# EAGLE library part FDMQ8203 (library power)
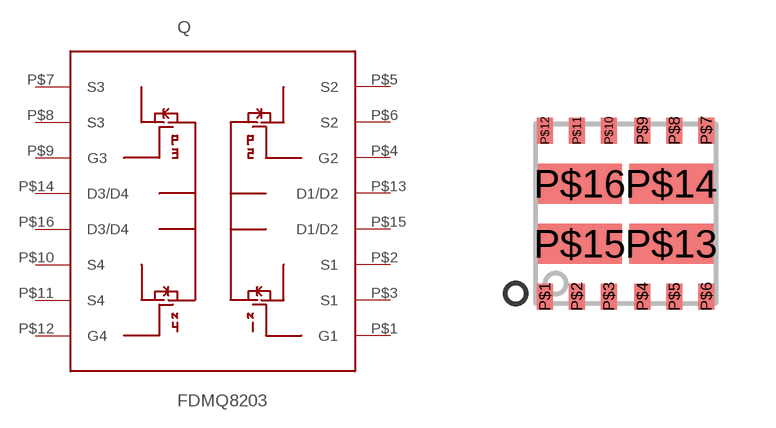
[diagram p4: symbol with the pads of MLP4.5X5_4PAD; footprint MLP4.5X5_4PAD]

Designator prefix Q

## FDMQ8203  [MLP4.5X5_4PAD]
P$1  G1
P$2  S1
P$3  S1
P$4  G2
P$5  S2
P$6  S2
P$7  S3
P$8  S3
P$9  G3
P$10  S4
P$11  S4
P$12  G4
P$13  D1/D2
P$14  D3/D4
P$15  D1/D2
P$16  D3/D4

## Footprint MLP4.5X5_4PAD (pad centres in mm)
smd 0.4 x 0.65: P$1 -2.02,-2.075; P$2 -1.22,-2.075; P$3 -0.42,-2.075; P$4 0.42,-2.075; P$5 1.22,-2.075; P$6 2.02,-2.075; P$7 2.02,2.075; P$8 1.22,2.075; P$9 0.42,2.075; P$10 -0.42,2.075; P$11 -1.22,2.075; P$12 -2.02,2.075
smd 2.1 x 1: P$13 1.142,-0.75; P$14 1.142,0.75; P$15 -1.142,-0.75; P$16 -1.142,0.75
